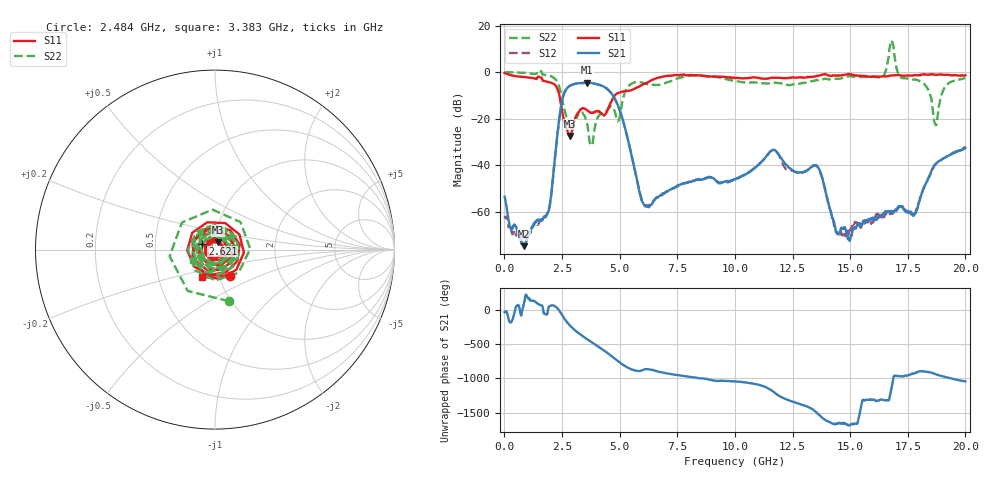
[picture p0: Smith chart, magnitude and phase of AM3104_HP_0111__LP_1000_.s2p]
!Created with skrf (http://scikit-rf.org).
# Hz S RI R 50.0
!freq ReS11 ImS11 ReS21 ImS21 ReS12 ImS12 ReS22 ImS22
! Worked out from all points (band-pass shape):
!   1601 points, 10 MHz to 20 GHz, reference 50 ohm
!   highest |S21| = -4.56 dB at 3.571 GHz (marker M1); lowest = -74.9 dB at 859.6 MHz (marker M2)
!   |S21| within 3 dB of the highest: 2.667 GHz to 4.509 GHz (1.842 GHz wide, 51.3 % of centre)
!   lowest |S11| = -27.4 dB at 2.859 GHz (marker M3), VSWR 1.09, Z = 51.3 + j4.12 ohm
!   |S11| at or under -10 dB: 2.386 GHz to 4.791 GHz (2.405 GHz wide, 67 % of centre)
!   |S22| runs from -31.3 to 13.7 dB; largest |S21 - S12| = 0.043
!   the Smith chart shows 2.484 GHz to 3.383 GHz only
!   S11 on the Smith chart (normalised r, x): 2.484 GHz: 1.13, -0.34; 2.621 GHz: 0.87, +0.06; 3.383 GHz: 0.83, -0.26
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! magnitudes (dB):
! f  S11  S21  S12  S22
! 10 MHz  -0.4  -53.6  -62.9  0.0
! 859.6 MHz  -2.1  -74.9  -71.2  -0.2
! 1.897 GHz  -4.2  -60.3  -60.2  -1.4
! 2.484 GHz  -15.5  -13.3  -13.3  -10.5
! 2.621 GHz  -22.2  -8.4  -8.4  -16.9
! 2.859 GHz  -27.4  -5.8  -5.8  -22.7
! 3.346 GHz  -15.8  -4.7  -4.7  -17.1
! 3.383 GHz  -15.5  -4.7  -4.7  -17.3
! 3.571 GHz  -16.3  -4.6  -4.6  -21.9
! 3.771 GHz  -17.5  -4.7  -4.7  -30.9
! 4.858 GHz  -9.4  -12.7  -12.8  -19.8
! 6.032 GHz  -5.2  -56.6  -56.5  -4.6
! 6.682 GHz  -2.4  -53.6  -53.7  -5.5
! 10.01 GHz  -2.5  -46.3  -46.2  -3.8
! 11.64 GHz  -2.4  -33.6  -33.5  -4.4
! 13.34 GHz  -2.1  -40.7  -40.7  -3.9
! 14.47 GHz  -1.6  -69.8  -69.6  -2.9
! 16.68 GHz  -1.6  -60.2  -60.5  7.3
! 17.8 GHz  -1.3  -61.0  -61.0  -3.1
! 18.7 GHz  -1.2  -39.6  -39.6  -22.6
! 19.14 GHz  -1.2  -36.7  -36.6  -6.2
! 20 GHz  -1.4  -32.6  -32.2  -2.6
